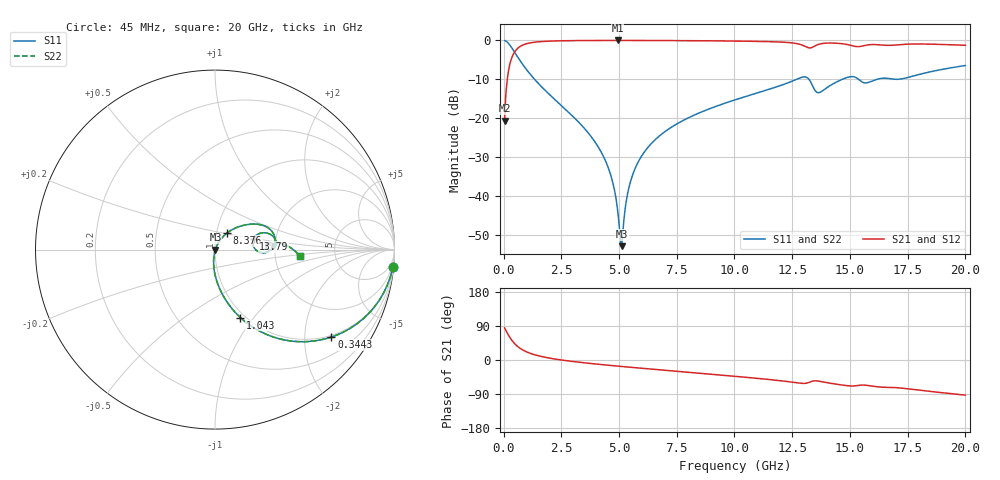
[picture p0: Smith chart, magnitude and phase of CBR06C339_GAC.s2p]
! S-parameter model data by Modelithics Inc.  support@modelithics.com 813-866-6335  Tampa FL USA
! S-Parameter data specifications:
! Substrate: 20-mil Rogers 4350B, substrate thickness, H=0.508mm, Dielectric constant, Er=3.75
! PCB Mounting Pad Footprint: Pad width, PadW=0.85mm , Pad length, PadL=0.64mm , Pad gap, PadG (edge-to-edge)=0.62mm , Reference planes=1.9mm apart
#  GHz  S  MA  R 50
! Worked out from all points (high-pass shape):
!   801 points, 45 MHz to 20 GHz, reference 50 ohm
!   highest |S21| = -0.02 dB at 4.934 GHz (marker M1); lowest = -20.6 dB at 45 MHz (marker M2)
!   |S21| within 3 dB of the highest: 475.2 MHz to end of sweep
!   lowest |S11| = -52.8 dB at 5.109 GHz (marker M3), VSWR 1.00, Z = 50.2 - j0.0233 ohm
!   |S11| at or under -10 dB: 1.343 GHz to 12.69 GHz (11.34 GHz wide, 162 % of centre); 13.22 GHz to 14.67 GHz (1.442 GHz wide, 10.3 % of centre); 15.37 GHz to 16.17 GHz (795.4 MHz wide, 5.04 % of centre)
!   |S22| runs from -52.8 to 0.0 dB; largest |S21 - S12| = 0
!   S11 on the Smith chart (normalised r, x): 45 MHz: 1, -21; 344.3 MHz: 0.95, -2.70; 1.043 GHz: 0.95, -0.86; 8.376 GHz: 1.12, +0.21; 13.79 GHz: 1.53, +0.19; 20 GHz: 2.79, -0.27
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0.045  0.9956 -5.5  0.09341 84.5  0.09341 84.5  0.9956 -5.5
0.194662  0.9263 -22.8  0.3764 67.2  0.3764 67.2  0.9263 -22.8
0.344325  0.8109 -36.9  0.5846 53.0  0.5846 53.0  0.8109 -36.9
0.668594  0.5763 -57.0  0.8164 32.9  0.8164 32.9  0.5763 -57.0
1.04275  0.4038 -69.5  0.9137 20.3  0.9137 20.3  0.4038 -69.5
3.387462  0.08087 -95.4  0.9947 -6.7  0.9947 -6.7  0.08087 -95.4
4.4351  0.02754 -98.9  0.9973 -13.2  0.9973 -13.2  0.02754 -98.9
4.734425  0.01479 -96.6  0.9975 -15.0  0.9975 -15.0  0.01479 -96.6
4.933975  0.006839 -87.3  0.9975 -16.1  0.9975 -16.1  0.006839 -87.3
5.03375  0.003345 -64.9  0.9975 -16.7  0.9975 -16.7  0.003345 -64.9
5.108581  0.002287 -5.8  0.9975 -17.1  0.9975 -17.1  0.002287 -5.8
5.382962  0.01121 59.5  0.9973 -18.6  0.9973 -18.6  0.01121 59.5
5.6324  0.02038 63.4  0.9971 -19.9  0.9971 -19.9  0.02038 63.4
6.704981  0.05791 61.8  0.9953 -25.6  0.9953 -25.6  0.05791 61.8
8.376212  0.114 54.1  0.9899 -34.3  0.9899 -34.3  0.114 54.1
10.0225  0.1724 45.6  0.9803 -43.0  0.9803 -43.0  0.1724 45.6
12.94092  0.3374 15.4  0.8678 -61.6  0.8678 -61.6  0.3374 15.4
13.36496  0.2672 -3.8  0.813 -56.0  0.813 -56.0  0.2672 -3.8
13.78901  0.2227 15.5  0.9109 -57.4  0.9109 -57.4  0.2227 15.5
14.98631  0.3406 9.7  0.8712 -68.3  0.8712 -68.3  0.3406 9.7
16.68248  0.3242 2.2  0.8625 -72.4  0.8625 -72.4  0.3242 2.2
20  0.4761 -4.4  0.8642 -92.7  0.8642 -92.7  0.4761 -4.4
